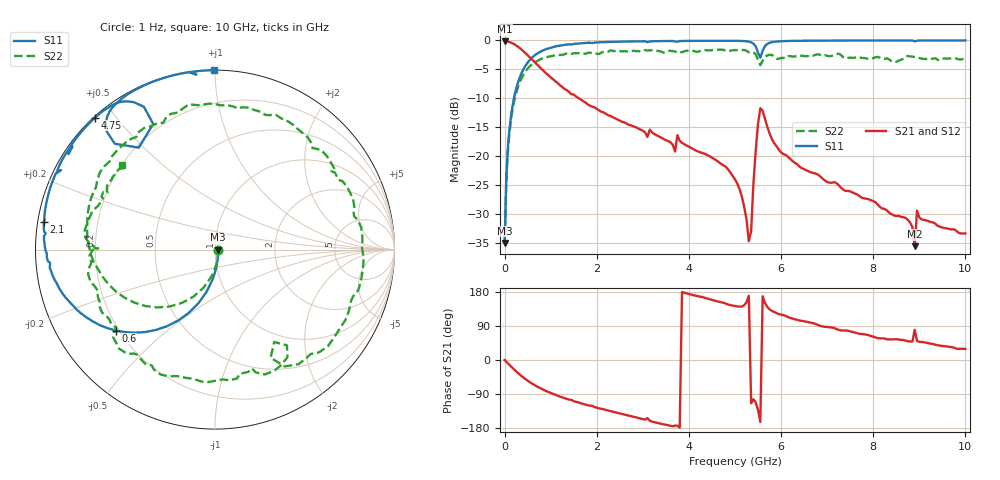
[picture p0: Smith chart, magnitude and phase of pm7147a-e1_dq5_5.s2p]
# GHz S DB R 50
! S-Parameters data
! Freq  dbS11  angS11  dbS21  angS21  dbS12  angS12  dbS22  angS22
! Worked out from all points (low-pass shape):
!   279 points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, 1 Hz to 10 GHz, reference 50 ohm
!   highest |S21| = -0.16 dB at 3.162 kHz (marker M1); lowest = -35.6 dB at 8.9 GHz (marker M2)
!   |S21| within 3 dB of the highest: start of sweep to 576.5 MHz
!   lowest |S11| = -35.0 dB at 2.512 kHz (marker M3), VSWR 1.04, Z = 51.8 - j0.000419 ohm
!   |S11| at or under -10 dB: start of sweep to 202 MHz
!   |S22| runs from -35.0 to -1.6 dB; largest |S21 - S12| = 0
!   S11 on the Smith chart (normalised r, x): 1 Hz: 1.04, -0.00; 600 MHz: 0.19, -0.35; 2.1 GHz: 0.02, +0.08; 4.75 GHz: 0.00, +0.44; 10 GHz: 0.00, +0.99
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1e-09  -35.04 -0.0  -0.16 -0.0  -0.16 -0.0  -35.04 -0.0
2.5119e-06  -35.04 -0.0  -0.16 -0.0  -0.16 -0.0  -35.04 -0.0
3.1623e-06  -35.04 -0.0  -0.16 -0.0  -0.16 -0.0  -35.04 -0.0
0.05011872  -21.51 -82.9  -0.19 -6.2  -0.19 -6.2  -22.19 -83.8
0.15  -12.38 -101.3  -0.42 -18.4  -0.42 -18.4  -13.09 -106.7
0.6  -2.94 -140.8  -3.34 -62.6  -3.34 -62.6  -4.10 -161.9
1.05  -1.15 -162.4  -6.71 -89.5  -6.71 -89.5  -2.64 163.8
1.7  -0.47 179.0  -10.48 -115.9  -10.48 -115.9  -2.23 127.1
2.1  -0.30 170.7  -12.35 -128.9  -12.35 -128.9  -2.10 110.3
3.35  -0.12 150.6  -16.61 -166.9  -16.61 -166.9  -1.82 50.3
4.75  -0.06 132.2  -21.61 151.0  -21.61 151.0  -1.63 -16.0
5.05  -0.07 127.8  -24.77 141.4  -24.77 141.4  -1.69 -31.3
5.3  -0.21 122.5  -34.74 169.4  -34.74 169.4  -2.06 -47.5
5.55  -2.98 126.8  -11.73 -163.7  -11.73 -163.7  -4.28 -57.4
5.7  -0.60 130.6  -14.90 140.2  -14.90 140.2  -2.60 -60.1
6.7  -0.04 115.6  -22.94 97.0  -22.94 97.0  -2.62 -107.5
7.3  -0.02 110.0  -25.49 78.0  -25.49 78.0  -2.52 -139.3
8.35  -0.01 101.5  -29.83 54.2  -29.83 54.2  -3.32 -179.7
8.8  -0.01 98.0  -31.51 48.7  -31.51 48.7  -2.77 168.9
8.9  -0.17 96.1  -35.60 79.6  -35.60 79.6  -2.87 164.3
8.95  -0.04 97.9  -29.44 50.6  -29.44 50.6  -2.90 162.8
10  -0.00 90.4  -33.40 29.1  -33.40 29.1  -3.12 137.7
